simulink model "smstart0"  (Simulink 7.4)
settings: Solver=ode45  StartTime=0.0  StopTime=12  MaxStep=1e-3  RelTol=1e-4  AbsTol=1e-4
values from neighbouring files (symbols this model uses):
  Bm = 0.10    (= 0.1)    [IMabc2.m]    (also in imabcparam.m = 0.01; IMabcrun0.m = 0.01; IMabcrun1.m = 0.001; IMcur0.m = 1e-06)
  H = 0.60    (= 0.6)    [IMabc2.m]    (also in IMcur0.m = 0.3; imdef0vec.m = 0.3; imdef1vec.m = 0.3; imdef2vec.m = 0.3)
  Ra = .95    (= 0.95)    [altwdgs.m]    (also in Ccurverun.m = 0.018)
  V = [Vas 0 0].'    [Actac.m]    (also in acttrcalc1.m = str2num(get(h,'string')); im3d.m = eval(get(hVs,'String')); IMabc2.m = [vas vbs vcs 0 0 0]'; IMabcf0.m = [vas vbs vcs 0 0 0]')
  wo = 2*pi*freq0    [calc0.m]    (also in IMabc2.m = 376.991118431; imabcparam.m = 376.991118431; IMabcrun0.m = 376.991118431; IMabcrun1.m = 376.991118431)
undefined symbols (not defined in the file or in its folder): Lal, Lfl, Lkdl, Lkql, Lmd, Lmq, Rf, Rfstart, Rkd, Rkq

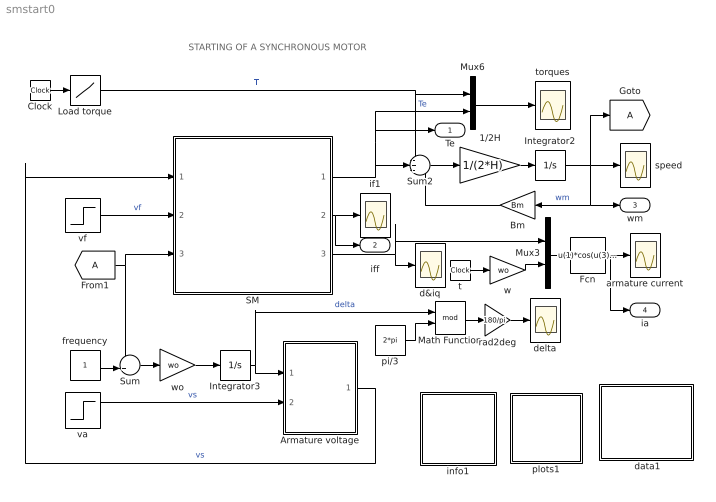
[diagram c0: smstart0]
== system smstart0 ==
  note: STARTING OF A SYNCHRONOUS MOTOR
  " data1" : Subsystem
  1/2H : Gain  Gain=1/(2*H)  ParameterDataType=sfix(16)  ParameterScaling=2^0  OutDataType=sfix(16)  OutScaling=2^0
  Armature voltage : Subsystem
  Bm : Gain  Gain=Bm  ParameterDataType=sfix(16)  ParameterScaling=2^0  OutDataType=sfix(16)  OutScaling=2^0
  Clock : Clock
  Fcn : Fcn  Expr=u(1)*cos(u(3))-u(2)*sin(u(3))
  Integrator2 : Integrator
  Integrator3 : Integrator
  Load torque : Lookup  InputValues=[0 10 10 30]  Table=[0.2 0.2 1 1]  OutDataType=sfix(16)  OutScaling=2^0
  Math Function : Math  Operator=mod
  Mux3 : Mux  Inputs=2
  Mux6 : Mux  Inputs=2
  SM : Subsystem
  Sum : Sum  Inputs=-+|  OutDataType=sfix(16)  OutScaling=2^0
  Sum2 : Sum  Inputs=-+-  OutDataType=sfix(16)  OutScaling=2^0
  armature current : Scope
  d&iq : Scope
  delta : Scope
  frequency : Constant  OutDataType=sfix(16)  OutScaling=2^0
  if1 : Scope
  info1 : Subsystem
  pi/3 : Constant  Value=2*pi  OutDataType=sfix(16)  OutScaling=2^0
  plots1 : Subsystem
  rad2deg : Gain  Gain=180/pi  ParameterDataType=sfix(16)  ParameterScaling=2^0  OutDataType=sfix(16)  OutScaling=2^0
  speed : Scope
  t : Clock
  torques : Scope
  va : Step  Time=0  After=V  SampleTime=0
  vf : Step  Time=5  After=0.02  SampleTime=0
  w : Gain  Gain=wo  ParameterDataType=sfix(16)  ParameterScaling=2^0  OutDataType=sfix(16)  OutScaling=2^0
  wo : Gain  Gain=wo  ParameterDataType=sfix(16)  ParameterScaling=2^0  OutDataType=sfix(16)  OutScaling=2^0
  Te : Outport
  iff : Outport  Port=2
  wm : Outport  Port=3
  ia : Outport  Port=4
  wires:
  Mux6/1 -> torques/1
  vf/1 -> SM/2(vf)  "vf"
  [A] -> SM/3(wm), Sum/1
  Sum2/1 -> 1/2H/1
  1/2H/1 -> Integrator2/1
  SM/1(Te) -> Sum2/2, Mux6/2, Te/1  "Te"
  Bm/1 -> Sum2/3
  Integrator2/1 -> speed/1, [A], Bm/1, wm/1  "wm"
  Armature voltage/1(vs) -> SM/1(vs)  "vs"
  SM/3(ia) -> d&iq/1, Mux3/1
  va/1 -> Armature voltage/2(Vt)  "vs"
  Integrator3/1 -> Armature voltage/1(delta), Math Function/1  "delta"
  frequency/1 -> Sum/2
  Sum/1 -> wo/1
  wo/1 -> Integrator3/1
  SM/2(if) -> if1/1, iff/1
  Math Function/1 -> rad2deg/1
  pi/3/1 -> Math Function/2
  rad2deg/1 -> delta/1
  w/1 -> Mux3/2
  Mux3/1 -> Fcn/1
  t/1 -> w/1
  Fcn/1 -> armature current/1, ia/1
  Clock/1 -> Load torque/1
  Load torque/1 -> Mux6/1, Sum2/1  "Tl"

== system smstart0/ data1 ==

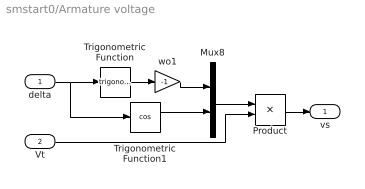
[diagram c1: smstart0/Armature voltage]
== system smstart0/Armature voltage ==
  delta : Inport  OutDataType=sfix(16)  OutScaling=2^0
  Vt : Inport  Port=2  OutDataType=sfix(16)  OutScaling=2^0
  Mux8 : Mux  Inputs=2
  Product : Product  OutDataType=sfix(16)  OutScaling=2^0
  Trigonometric Function : Trigonometry
  Trigonometric Function1 : Trigonometry  Operator=cos
  wo1 : Gain  Gain=-1  ParameterDataType=sfix(16)  ParameterScaling=2^0  OutDataType=sfix(16)  OutScaling=2^0
  vs : Outport
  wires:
  delta/1 -> Trigonometric Function/1, Trigonometric Function1/1
  Trigonometric Function/1 -> wo1/1
  Mux8/1 -> Product/1
  wo1/1 -> Mux8/1
  Trigonometric Function1/1 -> Mux8/2
  Product/1 -> vs/1
  Vt/1 -> Product/2

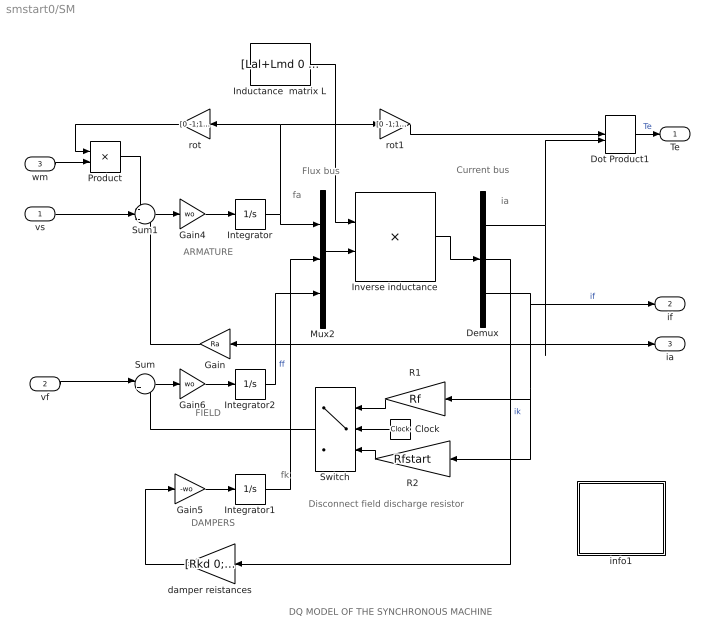
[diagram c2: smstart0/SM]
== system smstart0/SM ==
  note: DAMPERS
  note: ARMATURE
  note: fa
  note: fk
  note: ia
  note: FIELD
  note: DQ MODEL OF THE SYNCHRONOUS MACHINE
  note: Flux bus
  note: Current bus
  note: Disconnect field discharge resistor
  vs : Inport  OutDataType=sfix(16)  OutScaling=2^0
  vf : Inport  Port=2  OutDataType=sfix(16)  OutScaling=2^0
  wm : Inport  Port=3  OutDataType=sfix(16)  OutScaling=2^0
  Clock : Clock
  Demux : Demux  Outputs=3
  Dot Product1 : DotProduct  OutDataType=fixdt(1, 16)  OutScaling=2^-10
  Gain : Gain  Gain=Ra  ParameterDataType=sfix(16)  ParameterScaling=2^0  OutDataType=sfix(16)  OutScaling=2^0
  Gain4 : Gain  Gain=wo  ParameterDataType=sfix(16)  ParameterScaling=2^0  OutDataType=sfix(16)  OutScaling=2^0
  Gain5 : Gain  Gain=-wo  ParameterDataType=sfix(16)  ParameterScaling=2^0  OutDataType=sfix(16)  OutScaling=2^0
  Gain6 : Gain  Gain=wo  ParameterDataType=sfix(16)  ParameterScaling=2^0  OutDataType=sfix(16)  OutScaling=2^0
  Inductance  matrix L : Constant  Value=[Lal+Lmd 0 Lmd 0 Lmd;0 Lal+Lmq 0 Lmq 0;Lmd 0 Lmd+Lkdl 0 Lmd;0 Lmq 0 Lmq+Lkql 0;Lmd 0 Lmd 0 Lmd+Lfl]  VectorParams1D=off  OutDataType=fixdt(1, 16)  OutScaling=2^0
  Integrator : Integrator  InitialCondition=[0 0]
  Integrator1 : Integrator  InitialCondition=[0 0]
  Integrator2 : Integrator
  Inverse inductance : Product  Inputs=/*  Multiplication=Matrix(*)  OutDataType=sfix(16)  OutScaling=2^0
  Mux2 : Mux  Inputs=3
  Product : Product  OutDataType=sfix(16)  OutScaling=2^0
  R1 : Gain  Gain=Rf  ParameterDataType=sfix(16)  ParameterScaling=2^0  OutDataType=sfix(16)  OutScaling=2^0
  R2 : Gain  Gain=Rfstart  ParameterDataType=sfix(16)  ParameterScaling=2^0  OutDataType=sfix(16)  OutScaling=2^0
  Sum : Sum  Inputs=|+-  OutDataType=sfix(16)  OutScaling=2^0
  Sum1 : Sum  Inputs=-+-  OutDataType=sfix(16)  OutScaling=2^0
  Switch : Switch  Threshold=5
  damper reistances : Gain  Gain=[Rkd 0;0 Rkq]  Multiplication=Matrix(K*u)  ParameterDataType=sfix(16)  ParameterScaling=2^0  OutDataType=sfix(16)  OutScaling=2^0
  info1 : Subsystem
  rot : Gain  Gain=[0 -1;1 0]  Multiplication=Matrix(K*u)  ParameterDataType=sfix(16)  ParameterScaling=2^0  OutDataType=sfix(16)  OutScaling=2^0
  rot1 : Gain  Gain=[0 -1;1 0]  Multiplication=Matrix(K*u)  ParameterDataType=sfix(16)  ParameterScaling=2^0  OutDataType=sfix(16)  OutScaling=2^0
  Te : Outport
  if : Outport  Port=2
  ia : Outport  Port=3
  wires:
  Product/1 -> Sum1/1
  rot/1 -> Product/1
  wm/1 -> Product/2
  Gain5/1 -> Integrator1/1
  damper reistances/1 -> Gain5/1
  Integrator/1 -> Mux2/1, rot/1, rot1/1
  Sum1/1 -> Gain4/1
  Gain4/1 -> Integrator/1
  vs/1 -> Sum1/2
  Gain/1 -> Sum1/3
  Gain6/1 -> Integrator2/1
  Sum/1 -> Gain6/1
  vf/1 -> Sum/1
  rot1/1 -> Dot Product1/1
  Demux/1 -> Gain/1, ia/1, Dot Product1/2
  Dot Product1/1 -> Te/1  "Te"
  R2/1 -> Switch/3
  R1/1 -> Switch/1
  Clock/1 -> Switch/2
  Switch/1 -> Sum/2
  Integrator1/1 -> Mux2/2
  Integrator2/1 -> Mux2/3  "ff"
  Demux/3 -> if/1, R2/1, R1/1  "if"
  Demux/2 -> damper reistances/1  "ik"
  Mux2/1 -> Inverse inductance/2
  Inverse inductance/1 -> Demux/1
  Inductance  matrix L/1 -> Inverse inductance/1

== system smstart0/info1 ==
  note: Synchronous motor start
  note: Click the DATA block to enter and modify the parameters Initialize, Close, and then Start the simulation.

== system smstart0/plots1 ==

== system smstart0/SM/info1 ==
  note: This demonstration illustrates the dynamics of a synchronous generator, initially at no load, following a three-phase short circuit at the terminals.
  note: Synchronous machine transients under shortcircuit
